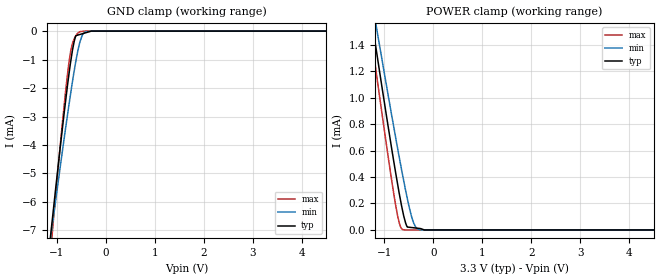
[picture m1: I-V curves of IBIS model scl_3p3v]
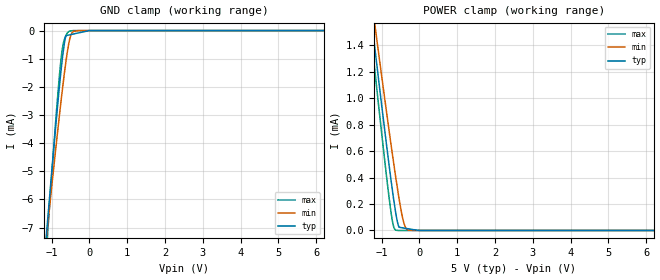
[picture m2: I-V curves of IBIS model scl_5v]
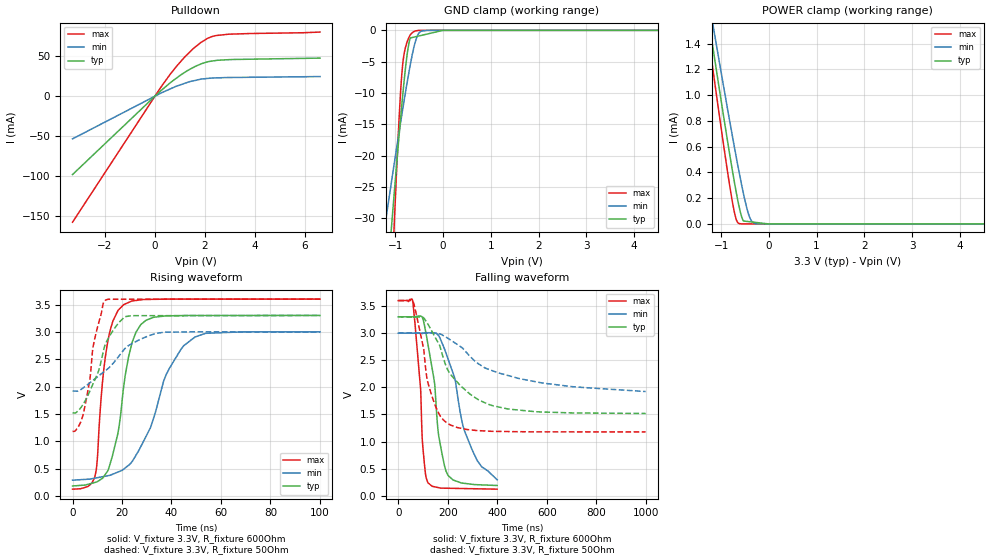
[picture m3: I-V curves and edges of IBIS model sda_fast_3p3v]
|Texas Instruments Incorporated
|Low-Power Rail-To-Rail Output 12-Bit I2C Input DAC
| Marketing part#   Digital Voltage Range   Package-type   #pins
| DAC7571IDBVR   2.7 to 5.5V   SOT-23   6
| DAC7571IDBVRG4   2.7 to 5.5V   SOT-23   6
| DAC7571IDBVRG4   2.7 to 5.5V   SOT-23   6
| DAC7571IDBVTG4   2.7 to 5.5V   SOT-23   6
[IBIS Ver]   3.2
[File name]   dac7571.ibs
|SIMDE Ver   V2.1 201006 Build 390
[File Rev]   1.1
[Date]   08/16/2010
[Source]
|   Texas Instruments Incorporated.
|   Analog-eLab Design Center, HPA
|   12500 TI Blvd
|   Dallas, TX -75243
|   e-mail: elab_ibis@list.ti.com
|   Model generated from simulations in SPECTRE
[Notes]   Revision History:
|   Rev 1.0: 08/02/2010
|   - Initial version of the model
|   - Model generated from simulations in SPECTRE
|   - Model matched to SPICE simulation
|   - Model names with a trailing 3p3v contains the model for
|   3.3V [3.0V and 3.6V]. Model names with trailing 5pv contains
|   the model for 5V [4.5V and 5.5V] operation.
|   - C_comp although listed in numerical order of value are obtained
|   from varying PVT conditions. For PVT conditions for each specific
|   value refer the buffer description under respective [Model]. IBIS
|   model user is responsible for using appropriate C_comp to simulate
|   for Signal Integrity.
|   Rev 1.1 : 08/16/2010
|   - Version 1.1 of the model
|   - Model generated from simulations in SPECTRE
|   - Model matched to SPECTRE simulation
|   - Changed the model for SDA from input to io open drain
|   - Model for A0 changed from NC to input(used the SCL model)
|   Rev 1.2 : 08/16/2010
|   - model_names changed to match signal_names
[Disclaimer]
| This model is designed as an aid for customers of Texas Instruments.
| TI and its licensors and suppliers make no warranties, either expressed
| or implied, with respect to this  model, including the warranties of
| merchantability or fitness for a particular purpose. The model is
| provided solely on an "as is" basis. The entire risk as to its quality
| and performance is with the customer.
[Copyright]
|(C) Copyright 2010 Texas Instruments Incorporated.All rights reserved.
|   DAC7571
[Component]   DAC7571
[Manufacturer]  TI
[Package]   | 6 SOT-23 - DBV package
|   typ   min   max
R_pkg   0.15948   0.15495   0.17131
L_pkg   4.45457nH   4.22280nH   4.76213nH
C_pkg   0.36982pF   0.35072pF   0.41205pF
[Pin]  signal_name  model_name   R_pin   L_pin   C_pin
1   VOUT   NC   0.15583   4.40388nH   0.36138pF
2   GND   GND   0.17136   5.69763nH   0.92603pF
3   VDD   POWER   0.15492   4.22624nH   0.34524pF
4   SDA   SDA   0.15495   4.22280nH   0.35072pF
5   SCL   SCL   0.17131   4.76213nH   0.41205pF
6   A0   A0   0.15582   4.42945nH   0.35514pF
[Model selector] SCL
 scl_3p3v   3.3V digital input
 scl_5v   5.0V digital input
[Model selector] A0
 a0_3p3v   3.3V digital input
 a0_5v   5.0V digital input
[Model selector] SDA
 sda_fast_3p3v   3.3V io open drain in fast mode(freq-3.4M,Rload=600ohm)
 sda_fast_5v   5.0V io open drain in fast mode(freq-3.4M,Rload=600ohm)
 sda_std_3p3v   3.3V io open drain in standard mode(freq-400k,Rload=2Kohm)
 sda_std_5v   5v io open drain in standard mode(freq-400k,Rload=2Kohm)
| Models and submodels in the file (8): scl_3p3v (Input), scl_5v (Input), a0_3p3v (Input), a0_5v (Input), sda_fast_3p3v (I/O_open_drain), sda_fast_5v (I/O_open_drain), sda_std_3p3v (I/O_open_drain), sda_std_5v (I/O_open_drain)
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|   INPUT SCL 3.3V Model
[Model]   scl_3p3v
Model_type   Input
Vinl = 0.99
Vinh = 2.31
|   typ   min   max
|   (nom PVT)   (Fast PVT)   (Slow PVT)
C_comp   4.196e-12   4.137e-12   4.262e-12
|Where nom PVT is NOM Process, 3.3V,25C
|   Fast PVT is Strong Process, 3.6V, -40C
|   Slow PVT is Weak Process, 3.0V, 105C
[Model spec]
|   typ   min   max
Vinl   0.99   0.9   1.08
Vinh   2.31   2.1   2.52
[Voltage Range]   3.3   3   3.6
|Junction Temperature
[Temperature Range]   25   105   -40
[Power Clamp Reference]   3.3   3   3.6
[GND Clamp Reference]   0   0   0
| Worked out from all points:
|   GND clamp passes 1 mA (typ) near -0.71 V on its own axis
|   POWER clamp passes 1 mA (typ) near -1.02 V on its own axis
[GND Clamp]
|   Voltage   I(typ)   I(min)   I(max)
-3.3V     -43.3mA    -36.41mA   -55.69mA
-1.142V   -7.355mA   -7.431mA   -8.009mA
-1.083V   -6.42mA    -6.666mA   -6.828mA
-888mV    -3.393mA   -4.196mA   -3.193mA
-790.8mV  -1.983mA   -3.009mA   -1.6mA
-740.4mV  -1.318mA   -2.413mA   -921.8uA
-686.4mV  -695.8uA   -1.8mA     -447.8uA
-630.3mV  -243uA     -1.211mA   -204.2uA
-524.4mV  -115uA     -342.4uA   -19.19uA
-453mV    -78.69uA   -71.83uA   -2.773uA
-297mV    0A         0A         0A
6.6V      0A         0A         0A
[POWER Clamp]
|   Voltage   I(typ)   I(min)   I(max)
-3.3V     6.65mA     6.278mA    7.032mA
-1.316V   1.72mA     1.862mA    1.585mA
-1.247V   1.552mA    1.712mA    1.401mA
-1.154V   1.327mA    1.509mA    1.152mA
-873.6mV  661.9uA    909.4uA    424.7uA
-762mV    410.8uA    677.8uA    166uA
-690mV    258.7uA    532.3uA    41.74uA
-621.6mV  130.9uA    398.7uA    2.09uA
-534.6mV  22.21uA    239.2uA    0A
-411mV    16.91uA    59.35uA    0A
-261mV    10.48uA    667.2nA    0A
6.6V      0A         0A         0A
|   INPUT SCL 5V MODEL
[Model]   scl_5v
Model_type   Input
Vinl = 1.5
Vinh = 3.5
|   typ   min   max
|   (nom PVT)   (Fast PVT)   (Slow PVT)
C_comp   4.159e-12   4.107e-12   4.214e-12
|Where nom PVT is NOM Process, 5.0V,25C
|   Fast PVT is Strong Process, 5.5V, -40C
|   Slow PVT is Weak Process, 4.5V, 105C
[Model spec]
|   typ   min   max
Vinl   1.5   1.35   1.65
Vinh   3.5   3.15   3.85
[Voltage Range]   5   4.5   5.5
|Junction Temperature
[Temperature Range]   25   105   -40
[Power Clamp Reference]   5   4.5   5.5
[GND Clamp Reference]   0   0   0
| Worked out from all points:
|   GND clamp passes 1 mA (typ) near -0.72 V on its own axis
|   POWER clamp passes 1 mA (typ) near -1.02 V on its own axis
[GND Clamp]
|   Voltage   I(typ)   I(min)   I(max)
-5V       -71.99mA   -59.56mA   -93.94mA
-1.153V   -7.505mA   -7.546mA   -8.189mA
-1.089V   -6.495mA   -6.736mA   -6.914mA
-875mV    -3.167mA   -4.015mA   -2.935mA
-798mV    -2.065mA   -3.081mA   -1.679mA
-737.5mV  -1.269mA   -2.359mA   -866.6uA
-688mV    -709.2uA   -1.807mA   -445.5uA
-620mV    -180.1uA   -1.101mA   -175.8uA
-528.5mV  -153.4uA   -353.8uA   -20.04uA
-459.5mV  -133.2uA   -81.14uA   -4.502uA
-288.5mV  -83.23uA   0A         0A
10V       0A         0A         0A
[POWER Clamp]
|   Voltage   I(typ)   I(min)   I(max)
-5V       10.91mA    10.1mA     11.74mA
-1.34V    1.773mA    1.91mA     1.644mA
-1.265V   1.591mA    1.746mA    1.442mA
-1.222V   1.485mA    1.652mA    1.325mA
-1.155V   1.324mA    1.508mA    1.149mA
-765mV    412.6uA    680.4uA    167.9uA
-688mV    250.4uA    525.7uA    36.76uA
-627.5mV  136.3uA    406uA      2.254uA
-540mV    24.35uA    244.8uA    0A
-450.5mV  20.14uA    104uA      0A
-306.5mV  13.37uA    3.888uA    0A
10V       0A         0A         0A
|   IO_OPEN DRAIN SDA 3.3V MODEL
|   3.3V fast mode, freq-3.4M,Rload=600ohm,  Cload = 15pF
[Model]   sda_fast_3p3v
Model_type   I/O_open_drain
Polarity   Non-Inverting
Enable   Active-Low
Vinl = 0.99
Vinh = 2.31
Vmeas = 1.65
Vref = 3.3
Cref = 15pF
Rref = 600
|   typ   min   max
|   (nom PVT)   (Fast PVT)   (Slow PVT)
|Average
C_comp   5.117e-12   5.087e-12   5.165e-12
|ON state : BUFFER OUTPUT TURNED LOW
|C_comp   8.694e-11   4.037e-11   1.679e-10
|OFF state : BUFFER IN HIGH IMPEDANCE STATE
|C_comp   5.117e-12   5.165e-12   5.087e-12
|Where nom PVT is NOM Process, 3.3V,25C
|   Fast PVT is Strong Process, 3.6V, -40C
|   Slow PVT is Weak Process, 3.0V, 105C
[Model spec]
|   typ   min   max
Vinl   0.99   0.9   1.08
Vinh   2.31   2.1   2.52
[Voltage Range]   3.3   3   3.6
|Junction temperature
[Temperature Range]   25   105   -40
[Pullup Reference]   3.3   3   3.6
[Pulldown Reference]   0   0   0
[Power Clamp Reference]   3.3   3   3.6
[GND Clamp Reference]   0   0   0
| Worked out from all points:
|   slope of the pulldown table from 0 to 0.495 V, typ, clamps not added: 36.2 ohm
|   GND clamp passes 1 mA (typ) near -0.56 V on its own axis
|   POWER clamp passes 1 mA (typ) near -1.02 V on its own axis
|   falling waveform, V_fixture 3.3V, R_fixture 600Ohm: 20-80 % time 51ns typ, 93.6ns min, 28.3ns max; typ from 3.3 V to 0.19 V
|   rising waveform, V_fixture 3.3V, R_fixture 600Ohm: 20-80 % time 6.86ns typ, 14ns min, 4.37ns max; typ from 0.18 V to 3.3 V
|   falling waveform, V_fixture 3.3V, R_fixture 50Ohm: 20-80 % time 143ns typ, 275ns min, 66.1ns max; typ from 3.3 V to 1.52 V
|   rising waveform, V_fixture 3.3V, R_fixture 50Ohm: 20-80 % time 8.68ns typ, 15.1ns min, 5.17ns max; typ from 1.52 V to 3.3 V
[Pulldown]
|   Voltage   I(typ)   I(min)   I(max)
-3.3V     -97.88mA   -53.33mA   -157.4mA
318mV     9.006mA    5.005mA    14.9mA
876mV     22.96mA    12.66mA    37.86mA
1.204V    29.99mA    16.21mA    49.42mA
1.52V     35.68mA    19.08mA    59.08mA
1.826V    40.06mA    21.19mA    66.83mA
2.266V    43.78mA    22.62mA    74.33mA
2.946V    45.58mA    23.31mA    77.37mA
6.6V      47.55mA    24.48mA    80.03mA
[GND Clamp]
|   Voltage   I(typ)   I(min)   I(max)
-3.3V     -246.7mA   -140.1mA   -463.1mA
-1.269V   -49.35mA   -33.72mA   -76.76mA
-1.208V   -43.43mA   -30.6mA    -65.2mA
-1.072V   -30.43mA   -23.65mA   -39.58mA
-1.047V   -28.13mA   -22.41mA   -35.08mA
-1.021V   -25.74mA   -21.13mA   -30.4mA
-916.8mV  -16.27mA   -15.97mA   -13.2mA
-844.8mV  -10.23mA   -12.5mA    -5.268mA
-719.4mV  -2.164mA   -6.811mA   -1.175mA
-618mV    -1.095mA   -2.867mA   -222.2uA
-330mV    -584.6uA   -3.168uA   -32.31nA
6.6V      0A         0A         0A
[POWER Clamp]
|   Voltage   I(typ)   I(min)   I(max)
-3.3V     6.651mA    6.278mA    7.033mA
-1.313V   1.712mA    1.855mA    1.577mA
-1.247V   1.552mA    1.712mA    1.401mA
-1.154V   1.327mA    1.51mA     1.152mA
-873.6mV  662.5uA    910uA      425.5uA
-762mV    411.2uA    678.4uA    166.8uA
-690mV    259.4uA    532.3uA    42.61uA
-621.6mV  131.7uA    399.4uA    2.885uA
-534.6mV  22.99uA    239.9uA    49.46nA
-411mV    17.67uA    60.06uA    38nA
-261mV    11.22uA    1.335uA    24.09nA
6.6V      0A         0A         0A
[Ramp]
R_load = 600
|   typ   min   max
dV/dt_r   1.87194/6.76213e-09   1.6281/1.40066e-08   2.08671/4.36689e-09
dV/dt_f   1.85389/5.02733e-08   1.62284/9.36000e-08   2.08542/2.81757e-08
[Falling Waveform]
V_fixture = 3.3V
V_fixture_min = 3V
V_fixture_max = 3.6V
R_fixture = 600Ohm
|   Time   V(typ)   V(min)   V(max)
0s        3.3V       3V         3.6V
59ns      3.3V       3V         3.583V
90.27ns   3.314V     3V         1.976V
98.16ns   3.28V      2.992V     970.2mV
119.1ns   2.82V      3.007V     251.3mV
147.2ns   2.067V     3.003V     165.8mV
163.7ns   1.101V     2.951V     150.1mV
199.7ns   390.6mV    2.544V     139.6mV
296.8ns   213.6mV    869mV      131.4mV
400ns     190mV      295.3mV    122.7mV
[Rising Waveform]
V_fixture = 3.3V
V_fixture_min = 3V
V_fixture_max = 3.6V
R_fixture = 600Ohm
|   Time   V(typ)   V(min)   V(max)
0s        180.1mV    286.5mV    122.2mV
9.032ns   244.3mV    323.3mV    351.6mV
13.95ns   436.6mV    365.8mV    2.745V
18.32ns   1.136V     434.6mV    3.386V
20.7ns    2.006V     489.1mV    3.499V
24.07ns   2.805V     627.8mV    3.565V
27.74ns   3.139V     912.7mV    3.586V
37.83ns   3.292V     2.216V     3.599V
49.56ns   3.299V     2.907V     3.6V
100ns     3.3V       3V         3.6V
[Falling Waveform]
V_fixture = 3.3V
V_fixture_min = 3V
V_fixture_max = 3.6V
R_fixture = 50Ohm
|   Time   V(typ)   V(min)   V(max)
0s        3.3V       3V         3.6V
60.09ns   3.295V     3V         3.582V
102.5ns   3.282V     3V         2.715V
114.2ns   3.206V     3V         2.222V
125.5ns   3.12V      3V         1.997V
164.1ns   2.8V       2.989V     1.516V
206.7ns   2.267V     2.887V     1.316V
326.7ns   1.765V     2.427V     1.201V
443.5ns   1.6V       2.218V     1.185V
1us       1.518V     1.923V     1.178V
[Rising Waveform]
V_fixture = 3.3V
V_fixture_min = 3V
V_fixture_max = 3.6V
R_fixture = 50Ohm
|   Time   V(typ)   V(min)   V(max)
0s        1.517V     1.917V     1.178V
4.275ns   1.672V     1.975V     1.486V
6.945ns   1.911V     2.065V     2.108V
8.113ns   2.03V      2.107V     2.666V
8.768ns   2.098V     2.13V      2.831V
12.44ns   2.639V     2.26V      3.523V
13.68ns   2.815V     2.304V     3.589V
21.31ns   3.278V     2.702V     3.596V
33.9ns    3.296V     2.972V     3.597V
100ns     3.3V       3V         3.6V
